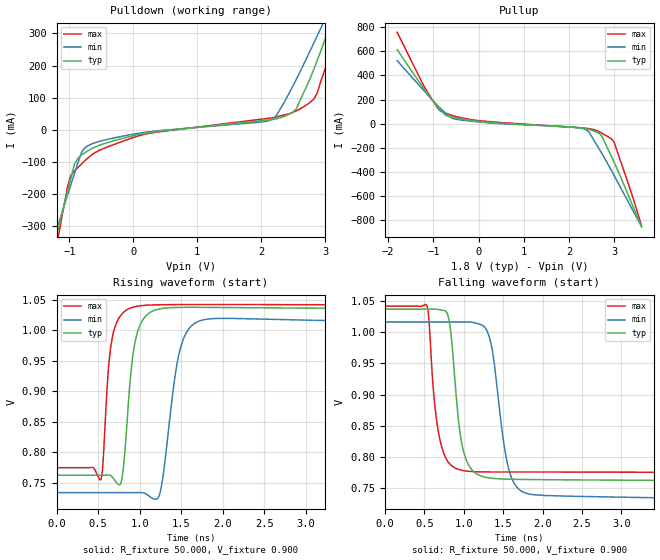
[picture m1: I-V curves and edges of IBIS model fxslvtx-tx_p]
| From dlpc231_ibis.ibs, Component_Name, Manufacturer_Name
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[Model] fxslvtx-tx_p
Model_type Output
Polarity   Non-Inverting
Vmeas =  0.900V
C_comp   4.596pF   4.567pF   4.628pF
C_comp_pullup   0.718pF   0.671pF   0.787pF
C_comp_pulldown   0.529pF   0.519pF   0.531pF
[Model Spec]
Vmeas   0.900V   0.900V   0.900V
[Temperature Range]   40.000   0.125k   -40.000
[Voltage Range]   1.800V   1.620V   1.980V
[Pullup Reference]   1.800V   1.620V   1.980V
[Pulldown Reference]   0.0V   0.0V   0.0V
[POWER Clamp Reference]   1.800V   1.620V   1.980V
[GND Clamp Reference]   0.0V   0.0V   0.0V
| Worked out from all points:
|   slope of the pulldown table from 0 to 0.27 V, typ, clamps not added: 26.4 ohm
|   slope of the pullup table from 0 to 0.27 V, typ, clamps not added: 26.3 ohm
|   rising waveform, R_fixture 50.000, V_fixture 0.900: 20-80 % time 115ps typ, 162ps min, 93.6ps max; typ from 0.763 V to 1.04 V
|   falling waveform, R_fixture 50.000, V_fixture 0.900: 20-80 % time 132ps typ, 177ps min, 123ps max; typ from 1.04 V to 0.763 V
[Pulldown]
|Voltage   I(typ)   I(min)   I(max)
-1.8V     -861.9mA   -731mA     -1.071A
-1.195V   -325.7mA   -310mA     -357.2mA
-975mV    -150.4mA   -170.7mA   -141.6mA
-700mV    -64.49mA   -48.72mA   -86.29mA
180mV     -11.16mA   -8.121mA   -13.74mA
2.105V    30.29mA    27.42mA    35.56mA
2.38V     43.45mA    93.62mA    47.16mA
2.545V    64.78mA    156.3mA    58.49mA
2.93V     245.8mA    316.5mA    151.1mA
3.095V    336.1mA    386mA      248.2mA
3.205V    397mA      432.4mA    324.4mA
3.6V      615.2mA    600.8mA    624mA
[Pullup]
|Voltage   I(typ)   I(min)   I(max)
-1.8V     614.6mA    523.2mA    759mA
-1.185V   275.8mA    263.9mA    296.7mA
-855mV    118.7mA    131.2mA    106.6mA
-745mV    73.55mA    92.03mA    88.76mA
-470mV    44.52mA    34.36mA    55.71mA
135mV     12.86mA    8.96mA     19.38mA
2.335V    -39.86mA   -46.08mA   -37.65mA
2.445V    -49.94mA   -73.94mA   -42.66mA
2.72V     -102.2mA   -245.9mA   -78.84mA
2.94V     -278.6mA   -394mA     -127.7mA
2.995V    -323.5mA   -432.3mA   -155.1mA
3.6V      -861.5mA   -855.2mA   -849.2mA
[Ramp]
| variable   typ   min   max
dV/dt_r   0.165/0.111n   0.169/0.152n   0.160/94.066p
dV/dt_f   0.165/0.140n   0.169/0.204n   0.160/0.123n
R_load = 50.000
[Rising Waveform]
R_fixture= 50.000
V_fixture= 0.900
V_fixture_min= 0.875
V_fixture_max= 0.908
|time   V(typ)   V(min)   V(max)
0s        762.5mV    734mV      774.9mV
536ps     762.5mV    734mV      756.5mV
642ps     762.6mV    734mV      961.8mV
772ps     748.8mV    734mV      1.025V
951ps     985mV      734.1mV    1.039V
1.217ns   1.035V     724.5mV    1.042V
1.437ns   1.038V     934.9mV    1.042V
1.517ns   1.038V     982.6mV    1.043V
1.936ns   1.038V     1.02V      1.043V
50ns      1.037V     1.016V     1.042V
[Falling Waveform]
R_fixture= 50.000
V_fixture= 0.900
V_fixture_min= 0.875
V_fixture_max= 0.908
|time   V(typ)   V(min)   V(max)
0s        1.037V     1.016V     1.042V
531ps     1.037V     1.016V     1.043V
653ps     1.037V     1.016V     861.3mV
785ps     1.031V     1.016V     795.3mV
985ps     815.4mV    1.016V     778.3mV
1.256ns   768mV      1.009V     775.9mV
1.356ns   765.8mV    975.5mV    775.8mV
1.596ns   764.2mV    770.2mV    775.8mV
2.046ns   763.5mV    738mV      775.8mV
50ns      762.5mV    734mV      774.9mV
